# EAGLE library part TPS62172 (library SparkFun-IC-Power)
Texas Instruments TPS62172 3-17V 0.5A Step-Down Converter with DCS control. Available in adjustable and fixed output voltage versions. Is packaged in an 8-pin WSON package measuring 2 × 2 mm (DSG). See a 3.3V fixed output version of this chip in action on the Electric Imp Breakout Board. Datasheet
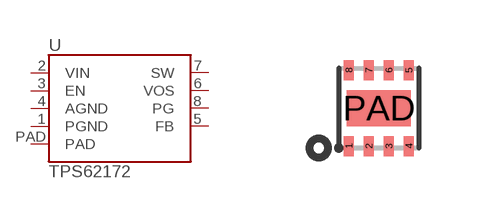
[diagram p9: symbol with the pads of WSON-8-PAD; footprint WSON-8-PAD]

Designator prefix U

## TPS62172 (PROD_ID: IC-11307)  [WSON-8-PAD]
1  PGND
2  VIN
3  EN
4  AGND
5  FB
6  VOS
7  SW
8  PG
PAD  PAD

## Footprint WSON-8-PAD (pad centres in mm)
smd 0.25 x 0.5: 1 -0.75,-0.95; 2 -0.25,-0.95; 3 0.25,-0.95; 4 0.75,-0.95; 5 0.75,0.95; 6 0.25,0.95; 7 -0.25,0.95; 8 -0.75,0.95
smd 1.6 x 0.9: PAD 0,0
